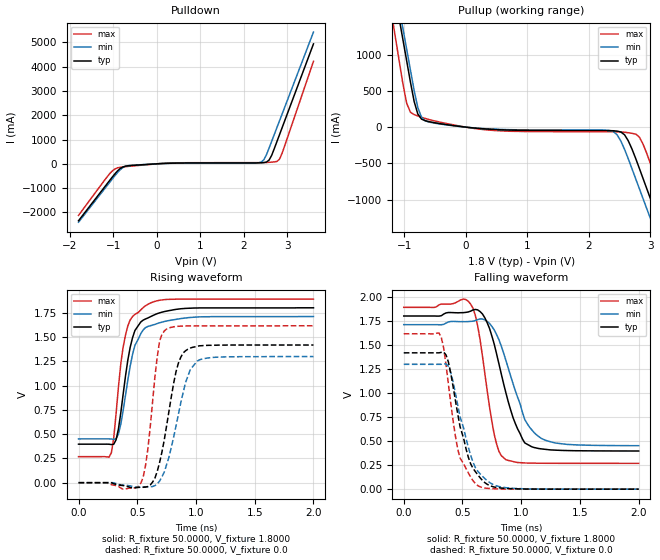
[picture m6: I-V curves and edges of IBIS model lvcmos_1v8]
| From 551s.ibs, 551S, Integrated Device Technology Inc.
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|   Model LVCMOS_1V8
[Model]   lvcmos_1v8
Model_type Output
Polarity   Non-Inverting
Vmeas =  0.9000V
Cref =   5.0000pF
Rref =   50.0000
Vref =   0.9000V
C_comp   2.0000pF   1.5000pF   2.5000pF
[Temperature Range]   55.0000   80.0000   -40.0000
[Voltage Range]   1.8000V   1.7100V   1.8900V
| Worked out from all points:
|   slope of the pulldown table from 0 to 0.27 V, typ, clamps not added: 12.1 ohm
|   slope of the pullup table from 0 to 0.27 V, typ, clamps not added: 12.4 ohm
|   rising waveform, R_fixture 50.0000, V_fixture 1.8000: 20-80 % time 112ps typ, 126ps min, 99.2ps max; typ from 0.396 V to 1.8 V
|   rising waveform, R_fixture 50.0000, V_fixture 0.0: 20-80 % time 124ps typ, 144ps min, 82.3ps max; typ from 0 V to 1.42 V
|   falling waveform, R_fixture 50.0000, V_fixture 1.8000: 20-80 % time 184ps typ, 202ps min, 119ps max; typ from 1.8 V to 0.397 V
|   falling waveform, R_fixture 50.0000, V_fixture 0.0: 20-80 % time 153ps typ, 164ps min, 120ps max; typ from 1.42 V to 0 V
[Pulldown]
|Voltage   I(typ)   I(min)   I(max)
-1.8V     -2.346A    -2.405A    -2.125A
-1.08V    -675.2mA   -752.9mA   -398.1mA
-900mV    -286mA     -351.9mA   -161.7mA
-720mV    -95.95mA   -100.9mA   -116.8mA
360mV     26.68mA    22.69mA    38.3mA
2.4V      43.84mA    72.17mA    49.31mA
2.46V     50.83mA    170mA      51.13mA
2.58V     154.9mA    650.6mA    61.35mA
2.64V     351.7mA    931.9mA    69.87mA
2.82V     1.203A     1.775A     194.7mA
2.88V     1.491A     2.056A     439.8mA
3.6V      4.942A     5.428A     4.223A
[Pullup]
|Voltage   I(typ)   I(min)   I(max)
-1.8V     4.939A     5.008A     4.686A
-1.2V     2.06A      2.194A     1.529A
-1.08V    1.484A     1.631A     898.3mA
-960mV    908.6mA    1.068A     326.9mA
-780mV    180.1mA    270mA      153.7mA
-240mV    25.77mA    22.91mA    37.68mA
2.4V      -50.22mA   -62.34mA   -64.36mA
2.76V     -432mA     -712.1mA   -95.85mA
3.06V     -1.127A    -1.4A      -648.3mA
3.18V     -1.405A    -1.676A    -939.5mA
3.36V     -1.823A    -2.089A    -1.376A
3.6V      -2.381A    -2.64A     -1.958A
[Ramp]
| variable   typ   min   max
dV/dt_r  0.8502/0.1243n   0.7788/0.1444n   0.9690/82.2548p
dV/dt_f  0.8420/0.1842n   0.7549/0.2218n   0.9731/0.1186n
R_load = 50.0000
[Rising Waveform]
R_fixture= 50.0000
V_fixture= 1.8000
V_fixture_min= 1.7100
V_fixture_max= 1.8900
|time   V(typ)   V(min)   V(max)
0s        396.3mV    450.9mV    268.1mV
280ps     392.2mV    449.6mV    310mV
300ps     395.8mV    445.5mV    462.7mV
340ps     555mV      501.6mV    988.5mV
400ps     1.099V     901.6mV    1.521V
440ps     1.395V     1.201V     1.676V
480ps     1.566V     1.413V     1.732V
570ps     1.685V     1.596V     1.821V
910ps     1.794V     1.695V     1.889V
2ns       1.8V       1.71V      1.89V
[Rising Waveform]
R_fixture= 50.0000
V_fixture= 0.0
V_fixture_min= 0.0
V_fixture_max= 0.0
|time   V(typ)   V(min)   V(max)
0s        0V         0V         0V
530ps     -46.45mV   -46.47mV   -5.854mV
590ps     -39.32mV   -43.2mV    343.8mV
650ps     46.03mV    -30.65mV   1.086V
690ps     207.2mV    16.71mV    1.457V
750ps     587.8mV    186.7mV    1.582V
850ps     1.23V      702.5mV    1.61V
910ps     1.357V     1.027V     1.613V
1.01ns    1.403V     1.25V      1.614V
2ns       1.417V     1.298V     1.615V
[Falling Waveform]
R_fixture= 50.0000
V_fixture= 1.8000
V_fixture_min= 1.7100
V_fixture_max= 1.8900
|time   V(typ)   V(min)   V(max)
0s        1.8V       1.71V      1.89V
570ps     1.851V     1.744V     1.923V
630ps     1.863V     1.763V     1.694V
710ps     1.731V     1.745V     1.027V
790ps     1.408V     1.608V     471mV
870ps     999.5mV    1.337V     305.2mV
930ps     745.3mV    1.098V     287.6mV
1.03ns    481.1mV    724.2mV    272.3mV
1.17ns    418.9mV    528.5mV    269.7mV
2ns       396.7mV    451.9mV    268.2mV
[Falling Waveform]
R_fixture= 50.0000
V_fixture= 0.0
V_fixture_min= 0.0
V_fixture_max= 0.0
|time   V(typ)   V(min)   V(max)
0s        1.417V     1.298V     1.615V
320ps     1.422V     1.298V     1.576V
340ps     1.425V     1.302V     1.466V
380ps     1.322V     1.278V     1.093V
460ps     778.7mV    871mV      414mV
550ps     330.9mV    434.5mV    168.9mV
630ps     149.5mV    187.1mV    37.95mV
730ps     37.9mV     69.72mV    6.973mV
870ps     8.203mV    15.54mV    1.279mV
2ns       62.01uV    71.84uV    47.62uV
